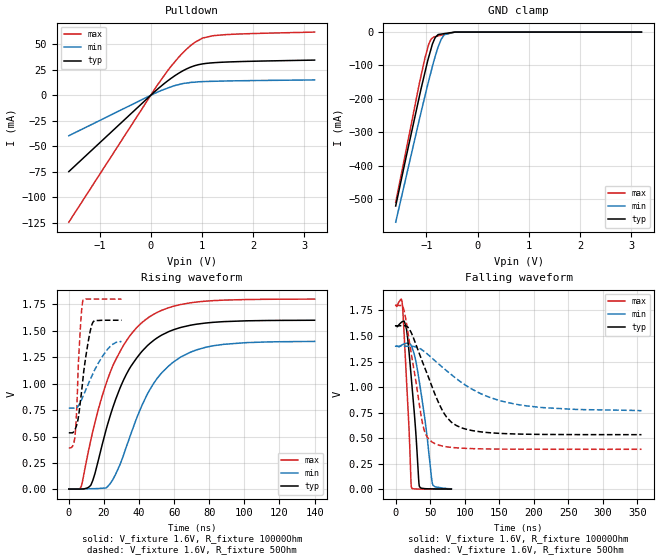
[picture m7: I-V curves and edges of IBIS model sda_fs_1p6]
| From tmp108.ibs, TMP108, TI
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|   sda_fs_1p6 Model
[Model]   sda_fs_1p6
Model_type   I/O_open_drain
Polarity   Non-Inverting
Vinl = 0.5
Vinh = 1.4
Vmeas = 0.8
Vref = 1.6
Cref = 2pF
Rref = 10000
|   typ   min   max
C_comp   9.450e-13   9.305e-13   9.710e-13
| Where nom  PVT is Nominal Process, 1.6V, 27C
|   Fast PVT is Strong Process,  1.8V, -40C
|   Slow PVT is Weak Process,   1.4V, 125C
[Voltage Range]   1.6   1.4   1.8
|Ambient Temperature   25   125   -40
|Junction Temperature
[Temperature Range]   27   125   -40
[Pullup Reference]   1.6   1.4   1.8
[Pulldown Reference]   0   0   0
[Power Clamp Reference]   1.6   1.4   1.8
[GND Clamp Reference]   0   0   0
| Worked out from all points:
|   slope of the pulldown table from 0 to 0.24 V, typ, clamps not added: 22.7 ohm
|   GND clamp passes 1 mA (typ) near -0.49 V on its own axis
|   falling waveform, V_fixture 1.6V, R_fixture 10000Ohm: 20-80 % time 11.1ns typ, 16.5ns min, 7.85ns max; typ from 1.6 V to 0.003 V
|   rising waveform, V_fixture 1.6V, R_fixture 10000Ohm: 20-80 % time 22.9ns typ, 23.8ns min, 23.1ns max; typ from 0.003 V to 1.6 V
|   falling waveform, V_fixture 1.6V, R_fixture 50Ohm: 20-80 % time 38.7ns typ, 83.7ns min, 19.9ns max; typ from 1.6 V to 0.535 V
|   rising waveform, V_fixture 1.6V, R_fixture 50Ohm: 20-80 % time 4.94ns typ, 11.3ns min, 2.31ns max; typ from 0.535 V to 1.6 V
[Pulldown]
|   Voltage   I(typ)   I(min)   I(max)
-1.6V     -74.82mA   -39.68mA   -124.5mA
126mV     5.698mA    2.974mA    9.698mA
394.2mV   16.52mA    8.24mA     28.27mA
612mV     23.57mA    11.31mA    40.9mA
777.6mV   27.6mA     12.64mA    48.7mA
862.2mV   29.08mA    12.86mA    51.96mA
1.008V    30.76mA    13.41mA    55.97mA
1.238V    31.97mA    13.74mA    58.55mA
1.699V    32.99mA    14.22mA    60.05mA
3.2V      34.52mA    15.06mA    61.98mA
[GND Clamp]
|   Voltage   I(typ)   I(min)   I(max)
-1.6V     -521mA     -569.6mA   -510mA
-1.132V   -189.1mA   -258mA     -150mA
-1.028V   -120.1mA   -191.1mA   -77.06mA
-955.8mV  -75.43mA   -146.4mA   -36.66mA
-909mV    -50.02mA   -118.5mA   -21.14mA
-880mV    -34.58mA   -101.3mA   -17.55mA
-828.8mV  -16.42mA   -72.81mA   -13.38mA
-771.2mV  -7.324mA   -44.62mA   -11.36mA
-711.2mV  -5.968mA   -21.37mA   -9.266mA
-651mV    -4.608mA   -7.937mA   -7.161mA
-428.4mV  -33.37uA   -90.99uA   -36.31uA
3.2V      0A         0A         0A
[POWER Clamp]
|   Voltage   I(typ)   I(min)   I(max)
-1.6V     0A         0A         0A
-1.598V   0A         0A         0A
3.2V      0A         0A         0A
[Ramp]
R_load = 10000
|   typ   min   max
dV/dt_r   0.95795/2.28955e-08   0.836583/2.36964e-08   1.07864/2.30492e-08
dV/dt_f   0.95795/1.11521e-08   0.836583/1.65934e-08   1.07864/7.86081e-09
[Falling Waveform]
V_fixture = 1.6V
V_fixture_min = 1.4V
V_fixture_max = 1.8V
R_fixture = 10000Ohm
|   Time   V(typ)   V(min)   V(max)
0s        1.6V       1.4V       1.8V
8.01ns    1.633V     1.408V     1.861V
9.69ns    1.641V     1.415V     1.805V
15.81ns   1.561V     1.43V      1.05V
19.16ns   1.357V     1.427V     614.7mV
22.74ns   1.079V     1.403V     20.85mV
34.47ns   26.95mV    1.044V     3.235mV
42.38ns   7.246mV    683.9mV    2.822mV
53.27ns   4.944mV    54.99mV    2.582mV
80.6ns    3.416mV    5.681mV    2.272mV
[Rising Waveform]
V_fixture = 1.6V
V_fixture_min = 1.4V
V_fixture_max = 1.8V
R_fixture = 10000Ohm
|   Time   V(typ)   V(min)   V(max)
0s        3.416mV    5.68mV     2.272mV
7.14ns    3.546mV    5.501mV    29.91mV
12.47ns   38.66mV    6.449mV    461.5mV
17.15ns   298.1mV    8.884mV    777.1mV
23.7ns    704mV      57.85mV    1.113V
32.76ns   1.088V     402.7mV    1.405V
44.65ns   1.358V     898.2mV    1.617V
57ns      1.493V     1.169V     1.719V
72.99ns   1.563V     1.321V     1.773V
140ns     1.6V       1.4V       1.8V
[Falling Waveform]
V_fixture = 1.6V
V_fixture_min = 1.4V
V_fixture_max = 1.8V
R_fixture = 50Ohm
|   Time   V(typ)   V(min)   V(max)
0s        1.6V       1.4V       1.8V
12.22ns   1.6V       1.4V       1.747V
22.39ns   1.535V     1.4V       1.337V
39.09ns   1.241V     1.36V      638.2mV
44.07ns   1.156V     1.334V     529.9mV
56.64ns   934.3mV    1.26V      447.9mV
80.35ns   659.3mV    1.124V     411.2mV
108.7ns   578.1mV    987.5mV    399.3mV
191.3ns   539.4mV    815mV      392.8mV
356ns     535.2mV    769.4mV    392.3mV
[Rising Waveform]
V_fixture = 1.6V
V_fixture_min = 1.4V
V_fixture_max = 1.8V
R_fixture = 50Ohm
|   Time   V(typ)   V(min)   V(max)
0s        535.1mV    769.1mV    392.3mV
3.47ns    563.9mV    767.6mV    496.2mV
4.35ns    601mV      770.8mV    706.6mV
5.26ns    664.5mV    786.1mV    1.113V
6.38ns    802.1mV    818.3mV    1.47V
8.02ns    1.04V      877.4mV    1.785V
11.05ns   1.398V     995.2mV    1.8V
13.89ns   1.585V     1.1V       1.8V
22.13ns   1.6V       1.327V     1.8V
30ns      1.6V       1.4V       1.8V
